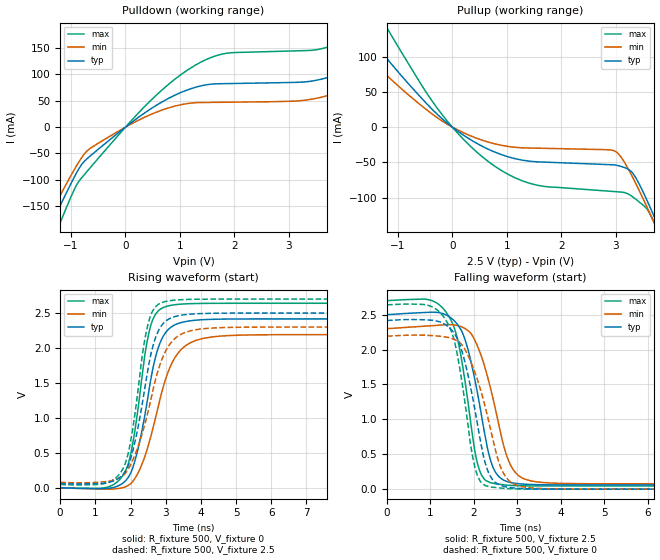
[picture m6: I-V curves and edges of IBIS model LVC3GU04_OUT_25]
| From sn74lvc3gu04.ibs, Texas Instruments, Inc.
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[Model]   LVC3GU04_OUT_25
Model_type  Output
Vref =   0
Rref =   500
Cref =   30p
Vmeas =   1.25
| variable   typ   min   max
C_comp   11.04pF   6.77pF   14.83pF
| C_pullup   11.53pF   6.99pF   14.57pF
| C_pulldown   10.56pF   6.77pF   14.83pF
[Temperature Range]   40   100   -40
| Ambient temperature   25   85   -40
[Voltage range]   2.5   2.3   2.7
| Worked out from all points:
|   slope of the pulldown table from 0 to 0.375 V, typ, clamps not added: 13.1 ohm
|   slope of the pullup table from 0 to 0.375 V, typ, clamps not added: 19.1 ohm
|   rising waveform, R_fixture 500, V_fixture 0: 20-80 % time 567ps typ, 748ps min, 457ps max; typ from 0 V to 2.42 V
|   falling waveform, R_fixture 500, V_fixture 2.5: 20-80 % time 468ps typ, 536ps min, 398ps max; typ from 2.5 V to 0.06 V
|   rising waveform, R_fixture 500, V_fixture 2.5: 20-80 % time 554ps typ, 742ps min, 455ps max; typ from 0.06 V to 2.5 V
|   falling waveform, R_fixture 500, V_fixture 0: 20-80 % time 471ps typ, 575ps min, 398ps max; typ from 2.42 V to 0 V
[Pulldown]
| LVC3GU04_OUT_25
|   Voltage   I(typ)   I(min)   I(max)
-5.5V     -1.065A    -962.2mA   -1.233A
-1.49V    -212.3mA   -186mA     -255.1mA
-1.26V    -162.1mA   -141.1mA   -196.6mA
-740mV    -63.16mA   -48.91mA   -88.2mA
-170mV    -14.05mA   -10.13mA   -19.98mA
910mV     60.77mA    39.99mA    91.21mA
1.805V    82.52mA    47.23mA    139.3mA
3.89V     99.97mA    65.23mA    158.5mA
4.44V     125.5mA    87.67mA    189.6mA
5.38V     188.7mA    141.4mA    271mA
6.09V     248.6mA    191.8mA    349.5mA
11V       818.3mA    670.6mA    1.103A
[Pullup]
| LVC3GU04_OUT_25
|   Voltage   I(typ)   I(min)   I(max)
-5.5V     592.1mA    472.8mA    820.6mA
-2.07V    183.1mA    140.6mA    261.6mA
-1.62V    137.2mA    104.3mA    197.4mA
-1.335V   109.5mA    82.71mA    158.4mA
-1.145V   91.71mA    68.9mA     133.2mA
-265mV    17.33mA    12.66mA    25.59mA
710mV     -33.04mA   -22.25mA   -51.52mA
1.55V     -49.14mA   -29.77mA   -82.08mA
2.995V    -53.62mA   -34.3mA    -91.33mA
3.32V     -65.79mA   -72.22mA   -99.02mA
3.77V     -137.9mA   -146.1mA   -147.1mA
11V       -1.614A    -1.516A    -1.794A
[Ramp]
| LVC3GU04_OUT_25
| variable   typ   min   max
dV/dt_r   1.46/5.75E-10   1.33/7.57E-10   1.59/4.63E-10
dV/dt_f   1.48/4.84E-10   1.37/5.59E-10   1.61/4.07E-10
R_load = 500
[Rising Waveform]
| LVC3GU04_OUT_25
R_fixture =   500
C_fixture =   0
L_fixture =   0
V_fixture =   0
V_fixture_min = 0
V_fixture_max = 0
|   Time   V(typ)   V(min)   V(max)
0s        34.4pV     5.528nV    1.802nV
1.325ns   -10.13mV   -20.11mV   5.937mV
1.815ns   78.82mV    5.697mV    200.2mV
2.165ns   458.4mV    166.8mV    953.8mV
2.56ns    1.503V     703.1mV    2.294V
2.805ns   2.028V     1.197V     2.539V
3.11ns    2.281V     1.709V     2.606V
3.69ns    2.388V     2.071V     2.634V
4.86ns    2.414V     2.179V     2.64V
24.99ns   2.416V     2.191V     2.64V
[Falling Waveform]
| LVC3GU04_OUT_25
R_fixture =   500
C_fixture =   0
L_fixture =   0
V_fixture =   2.5
V_fixture_min = 2.3
V_fixture_max = 2.7
|   Time   V(typ)   V(min)   V(max)
0s        2.5V       2.3V       2.7V
1.135ns   2.532V     2.345V     2.67V
1.645ns   2.338V     2.339V     2.09V
1.845ns   2.042V     2.279V     1.332V
2.08ns    1.383V     2.053V     374.4mV
2.305ns   606.1mV    1.63V      115.8mV
2.47ns    271.9mV    1.216V     80.26mV
2.89ns    89.24mV    293.7mV    52.57mV
3.6ns     62.77mV    94.57mV    46.03mV
24.99ns   60.06mV    77.04mV    45.59mV
[Rising Waveform]
| LVC3GU04_OUT_25
R_fixture =   500
C_fixture =   0
L_fixture =   0
V_fixture =   2.5
V_fixture_min = 2.3
V_fixture_max = 2.7
|   Time   V(typ)   V(min)   V(max)
0s        60.06mV    77.04mV    45.59mV
1.275ns   67.79mV    86.31mV    61.39mV
1.76ns    175mV      162.7mV    249.9mV
2.095ns   589.4mV    431.8mV    949.7mV
2.51ns    1.737V     1.113V     2.365V
2.73ns    2.173V     1.584V     2.599V
3.015ns   2.39V      1.972V     2.668V
3.53ns    2.475V     2.218V     2.693V
4.64ns    2.498V     2.292V     2.7V
24.99ns   2.5V       2.3V       2.7V
[Falling Waveform]
| LVC3GU04_OUT_25
R_fixture =   500
C_fixture =   0
L_fixture =   0
V_fixture =   0
V_fixture_min = 0
V_fixture_max = 0
|   Time   V(typ)   V(min)   V(max)
0s        2.416V     2.191V     2.64V
950ps     2.422V     2.202V     2.632V
1.38ns    2.341V     2.176V     2.394V
1.61ns    2.168V     2.125V     1.951V
2.03ns    1.113V     1.659V     297.8mV
2.215ns   485.4mV    1.285V     71.29mV
2.375ns   188.3mV    880.1mV    33.26mV
2.735ns   33.98mV    175.1mV    10.18mV
3.425ns   2.933mV    13.56mV    567.3uV
24.99ns   3.866nV    13.37nV    3.391nV
